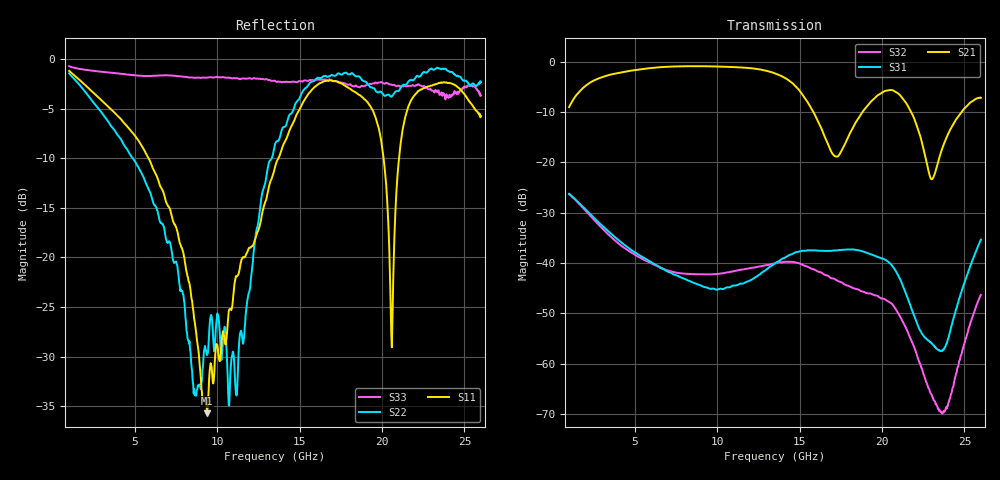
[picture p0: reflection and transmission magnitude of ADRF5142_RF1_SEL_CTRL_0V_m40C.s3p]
! Device: ADRF5142
! Description: Silicon, SPDT Switch, Reflective
! Frequency: 8.00 GHz - 11.00 GHz
! Ports:
!  RFC = Port 1
!  RF1 = Port 2
!  RF2 = Port 3
! VDD = +3.3V
! VSS = -3.3V
! CTRL = 0V
! Temp = -40C
! Data:  Data was collected using an calibrated 4 port network analyzer.
!  The reference plane is the package pins of ADRF5142 switch.
! Notes: Analog Devices supplies this data as a sample of measured data
!  for this product.  Your particular data for this product may vary.
!  Data was taken at -40 degrees C.
!  Analog Devices reserves the right to change this data at anytime.
# HZ S DB R 50
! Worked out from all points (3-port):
!   801 points, 1 GHz to 26 GHz, reference 50 ohm
!   strongest paths, dB at 1 GHz, 7.25 GHz, 13.5 GHz, 19.75 GHz, 26 GHz:
!     S21: -9.1, -1.0, -2.4, -6.7, -7.2
!     S31: -26.3, -42.1, -40.1, -38.8, -35.4
!     S32: -26.3, -41.7, -40.1, -46.6, -46.4
!   lowest |S11| = -35.7 dB at 9.375 GHz (marker M1), VSWR 1.03, Z = 48.8 + j1.14 ohm
!   |S11| at or under -10 dB: 5.823 GHz to 13.7 GHz (7.882 GHz wide, 80.7 % of centre); 20.09 GHz to 21.03 GHz (937.3 MHz wide, 4.56 % of centre)
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1e9  -1.19 158.5  -9.05 38.9  -26.29 -41.9
     -9.05 38.9  -1.44 123.8  -26.33 -60.5
     -26.29 -41.9  -26.33 -60.5  -0.72 169.3
2.875e9  -4.00 130.7  -3.26 -16.1  -32.22 -89.2
         -3.26 -16.1  -5.19 34.9  -32.70 -142.8
         -32.22 -89.2  -32.70 -142.8  -1.27 152.9
5.9062e9  -10.27 95.3  -1.32 -88.0  -39.70 -120.9
          -1.32 -88.0  -13.39 -77.0  -39.95 136.3
          -39.70 -120.9  -39.95 136.3  -1.70 127.8
9.375e9  -35.71 134.7  -0.95 -166.9  -44.92 -136.6
         -0.95 -166.9  -29.84 79.4  -42.30 63.4
         -44.92 -136.6  -42.30 63.4  -1.87 98.0
1.35e10  -10.90 -99.6  -2.37 88.2  -40.07 -153.0
         -2.37 88.2  -8.61 53.9  -40.11 -36.9
         -40.07 -153.0  -40.11 -36.9  -2.19 64.5
1.78125e10  -2.78 149.3  -15.94 74.9  -37.36 112.7
            -15.94 74.9  -1.37 -89.8  -44.44 176.5
            -37.36 112.7  -44.44 176.5  -2.54 23.0
2.05937e10  -29.06 -49.5  -5.67 0.3  -40.51 37.0
            -5.67 0.3  -3.75 -142.4  -48.13 62.2
            -40.51 37.0  -48.13 62.2  -2.60 -7.0
2.20312e10  -3.52 164.9  -12.04 -61.1  -51.21 19.2
            -12.04 -61.1  -1.87 -159.2  -57.48 -9.9
            -51.21 19.2  -57.48 -9.9  -2.64 -24.4
2.36875e10  -2.38 87.5  -16.97 13.3  -57.33 108.0
            -16.97 13.3  -0.98 163.3  -69.86 -89.3
            -57.33 108.0  -69.86 -89.3  -3.62 -48.7
2.6e10  -5.75 -1.0  -7.20 -40.5  -35.40 145.5
        -7.20 -40.5  -2.34 106.2  -46.37 128.1
        -35.40 145.5  -46.37 128.1  -3.67 -55.1
